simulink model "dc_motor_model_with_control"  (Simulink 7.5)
settings: Solver=ode45  StartTime=0.0  StopTime=20  RelTol=1e-3
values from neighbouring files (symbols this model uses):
  K = 12/4000    (= 0.003)    [INITIAL_PARAM.m]
  k2 = 12/4000    (= 0.003)    [INITIAL_PARAM.m]
  R = 10    [INITIAL_PARAM.m]
libraries: fl_lib x10, nesl_utility x4, simulink x1

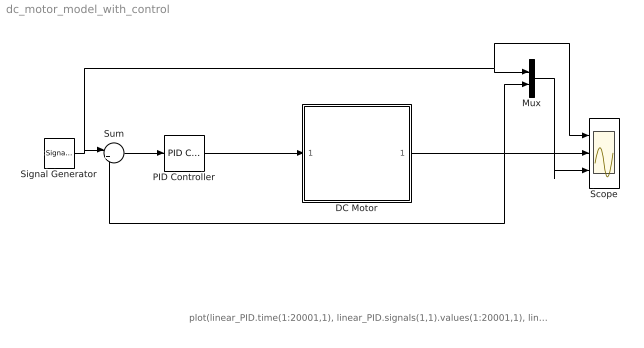
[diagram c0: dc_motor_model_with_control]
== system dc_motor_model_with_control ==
  note: plot(linear_PID.time(1:20001,1), linear_PID.signals(1,1).values(1:20001,1), linear_PID.time(1:20001,1),linear_PID.signals(1,2).values(1:20001,1)) >> grid on; >> title('Speed Response'); >> xlabel('Time in seconds'); >> ylabel('Speed in rpm'); >>
  DC Motor : Subsystem  mask{IMG='dcimaag.bmp'}
      mask prompts: IMG "Image File"
      mask init:
      | block=gcb;
      | img=imread(IMG);
  Mux : Mux  Inputs=2
  PID Controller : simulink/Continuous/PID Controller  DialogController=pidpack.PIDConfig.pidDDGCreate  DialogControllerArgs=DataTag0  SystemSampleTime=-1  Controller=PID  TimeDomain=Discrete-time  SampleTime=0.001  IntegratorMethod=Forward Euler  FilterMethod=Forward Euler  Form=Parallel  P=3.83525437608807  I=1.98635813727714  D=-1.09795088923682  N=3.48611026766055  InitialConditionSource=internal  InitialConditionForIntegrator=0  InitialConditionForFilter=0  ExternalReset=none  LimitOutput=off  UpperSaturationLimit=inf  LowerSaturationLimit=-inf  LinearizeAsGain=off  AntiWindupMode=none  Kb=1  TrackingMode=off  Kt=1  PParamMin=[]  PParamMax=[]  IParamMin=[]  IParamMax=[]  DParamMin=[]  DParamMax=[]  NParamMin=[]  NParamMax=[]  KbParamMin=[]  KbParamMax=[]  KtParamMin=[]  KtParamMax=[]  POutMin=[]  POutMax=[]  IOutMin=[]  IOutMax=[]  DOutMin=[]  DOutMax=[]  NOutMin=[]  NOutMax=[]  KbOutMin=[]  KbOutMax=[]  KtOutMin=[]  KtOutMax=[]  IntegratorOutMin=[]  IntegratorOutMax=[]  FilterOutMin=[]  FilterOutMax=[]  SumOutMin=[]  SumOutMax=[]  SumI1OutMin=[]  SumI1OutMax=[]  SumI2OutMin=[]  SumI2OutMax=[]  SumI3OutMin=[]  SumI3OutMax=[]  SumDOutMin=[]  SumDOutMax=[]  SaturationOutMin=[]  SaturationOutMax=[]  IntegratorContinuousStateAttributes=''  IntegratorStateMustResolveToSignalObject=off  IntegratorRTWStateStorageClass=Auto  FilterContinuousStateAttributes=''  FilterStateMustResolveToSignalObject=off  FilterRTWStateStorageClass=Auto
  Scope : Scope  NumInputPorts=3
  Signal Generator : SignalGenerator  WaveForm=square  Amplitude=2700  Frequency=1/10
  Sum : Sum  Inputs=|+-  OutDataType=fixdt(1, 16)  OutScaling=2^0
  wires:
  Signal Generator/1 -> Sum/1, Mux/1, Scope/1
  Sum/1 -> PID Controller/1
  PID Controller/1 -> DC Motor/1(Voltage)
  DC Motor/1(Speed) -> Scope/2, Mux/2, Sum/2
  Mux/1 -> Scope/3

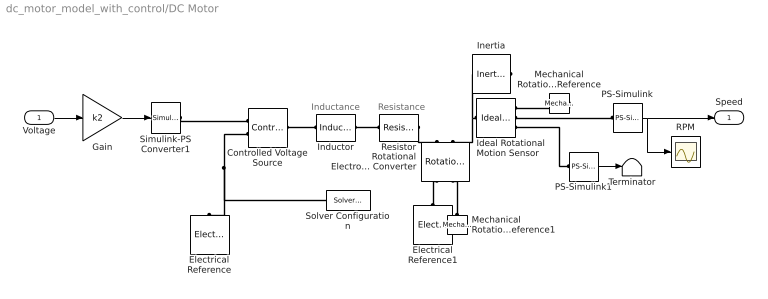
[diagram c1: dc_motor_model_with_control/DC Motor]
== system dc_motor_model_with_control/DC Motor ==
  note: Inductance
  note: Resistance
  Voltage : Inport  OutDataType=fixdt(1, 16)  OutScaling=2^0
  Controlled Voltage Source : fl_lib/Electrical/Electrical Sources/Controlled Voltage Source  DialogController=NetworkEngine.DynNeDlgSource  SystemSampleTime=-1  i_Log=off  v_Log=off  LocalVarNames=|i|v  LocalVarDescs=|i|v  LocalVarLogging=[0 0]
  Electrical Reference : fl_lib/Electrical/Electrical Elements/Electrical Reference  DialogController=NetworkEngine.DynNeDlgSource  SystemSampleTime=-1  i_Log=off  LocalVarNames=|i  LocalVarDescs=|i  LocalVarLogging=0
  Electrical Reference1 : fl_lib/Electrical/Electrical Elements/Electrical Reference  DialogController=NetworkEngine.DynNeDlgSource  SystemSampleTime=-1  i_Log=off  LocalVarNames=|i  LocalVarDescs=|i  LocalVarLogging=0
  Gain : Gain  Gain=k2  ParameterDataType=fixdt(1, 16)  ParameterScaling=2^0  OutDataType=fixdt(1, 16)  OutScaling=2^0
  Ideal Rotational Motion Sensor : fl_lib/Mechanical/Mechanical Sensors/Ideal Rotational Motion Sensor  DialogController=NetworkEngine.DynNeDlgSource  SystemSampleTime=-1  offset=0 deg  w_Log=off  t_Log=off  phi_Log=off  LocalVarNames=|w|t|phi  LocalVarDescs=|w|t|phi  LocalVarLogging=[]
  Inductor : fl_lib/Electrical/Electrical Elements/Inductor  DialogController=NetworkEngine.DynNeDlgSource  SystemSampleTime=-1  l=L mH  i0=0 A  r=0 Ohm  g=1e-9 1/Ohm  i_Log=off  v_Log=off  i_L_Log=off  LocalVarNames=|i|v|i_L  LocalVarDescs=|i|v|Internal variable for current through inductor term  LocalVarLogging=[0 0 0]
  Inertia : fl_lib/Mechanical/Rotational Elements/Inertia  DialogController=NetworkEngine.DynNeDlgSource  SystemSampleTime=-1  inertia=I kg*m^2  initial_velocity=0 rad/s  t_Log=off  LocalVarNames=|t  LocalVarDescs=|t  LocalVarLogging=0
  Mechanical Rotational Reference : fl_lib/Mechanical/Rotational Elements/Mechanical Rotational Reference  DialogController=NetworkEngine.DynNeDlgSource  SystemSampleTime=-1  t_Log=off  LocalVarNames=|t  LocalVarDescs=|t  LocalVarLogging=[]
  Mechanical Rotational Reference1 : fl_lib/Mechanical/Rotational Elements/Mechanical Rotational Reference  DialogController=NetworkEngine.DynNeDlgSource  SystemSampleTime=-1  t_Log=off  LocalVarNames=|t  LocalVarDescs=|t  LocalVarLogging=[]
  PS-Simulink : nesl_utility/PS-Simulink Converter  DialogController=NetworkEngine.DynNeUtilDlgSource  SystemSampleTime=-1  PhysicalDomain=network_engine_domain  LeftPortType=input  RightPortType=output  SubClassName=ps_output  Unit=rpm  AffineConversion=off
  PS-Simulink1 : nesl_utility/PS-Simulink Converter  DialogController=NetworkEngine.DynNeUtilDlgSource  SystemSampleTime=-1  PhysicalDomain=network_engine_domain  LeftPortType=input  RightPortType=output  SubClassName=ps_output  Unit=1  AffineConversion=off
  RPM : Scope
  Resistor : fl_lib/Electrical/Electrical Elements/Resistor  DialogController=NetworkEngine.DynNeDlgSource  SystemSampleTime=-1  R=R Ohm  i_Log=off  v_Log=off  LocalVarNames=|i|v  LocalVarDescs=|i|v  LocalVarLogging=[0 0]
  Rotational Electromechanical Converter : fl_lib/Electrical/Electrical Elements/Rotational Electromechanical Converter  DialogController=NetworkEngine.DynNeDlgSource  SystemSampleTime=-1  K=K V/rpm  i_Log=off  v_Log=off  t_Log=off  w_Log=off  LocalVarNames=|i|v|t|w  LocalVarDescs=|i|v|t|w  LocalVarLogging=[0 0 0 0]
  Simulink-PS Converter1 : nesl_utility/Simulink-PS Converter  DialogController=NetworkEngine.DynNeUtilDlgSource  SystemSampleTime=-1  PhysicalDomain=network_engine_domain  LeftPortType=input  RightPortType=output  SubClassName=ps_input  Unit=V  AffineConversion=off  InputFilterTimeConstant=.001  UdotUserProvided=0
  Solver Configuration : nesl_utility/Solver Configuration  DialogController=NetworkEngine.DynNeUtilDlgSource  SystemSampleTime=-1  PhysicalDomain=network_engine_domain  LeftPortType=input  RightPortType=generic  SubClassName=solver  Accelerate=off  Profile=off  ResidualTolerance=1e-9  MaxNonlinIter=3  MaxModeIter=2  DoFixedCost=off  UseLocalSampling=off  DoDC=off  LinearAlgebra=Sparse  LocalSolverSampleTime=.001  LocalSolverChoice=NE_BACKWARD_EULER_ADVANCER  UseLocalSolver=off
  Terminator : Terminator
  Speed : Outport  OutDataType=fixdt(1, 16)  OutScaling=2^0
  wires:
  PS-Simulink1/1 -> Terminator/1
  Voltage/1 -> Gain/1
  Gain/1 -> Simulink-PS Converter1/1
  PS-Simulink/1 -> Speed/1, RPM/1
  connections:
  Ideal Rotational Motion Sensor/LConn1 -- Rotational Electromechanical Converter/LConn2 -- Inertia/LConn1
  Inductor/RConn1 -- Resistor/LConn1
  Resistor/RConn1 -- Rotational Electromechanical Converter/LConn1
  PS-Simulink1/LConn1 -- Ideal Rotational Motion Sensor/RConn3
  Controlled Voltage Source/LConn1 -- Inductor/LConn1
  Simulink-PS Converter1/RConn1 -- Controlled Voltage Source/RConn1
  Electrical Reference1/LConn1 -- Rotational Electromechanical Converter/RConn1
  PS-Simulink/LConn1 -- Ideal Rotational Motion Sensor/RConn2
  Controlled Voltage Source/RConn2 -- Electrical Reference/LConn1 -- Solver Configuration/RConn1
  Mechanical Rotational Reference/LConn1 -- Ideal Rotational Motion Sensor/RConn1
  Mechanical Rotational Reference1/LConn1 -- Rotational Electromechanical Converter/RConn2
